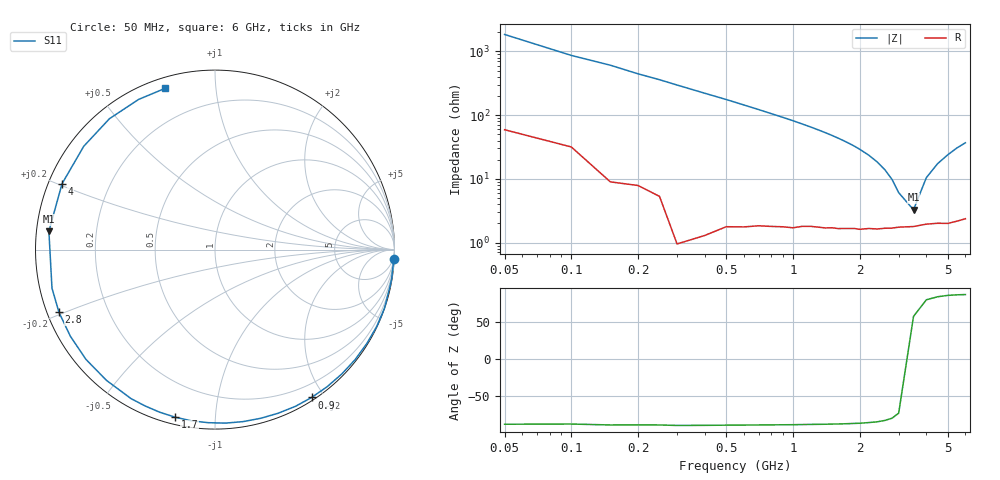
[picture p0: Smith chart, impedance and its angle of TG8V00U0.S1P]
! SIEMENS Discrete & RF Semiconductors
! BAT64
! Si Schottky Diode in SOT23
! VR = 8 V
! S-Parameters:  February  1997
# GHz  S  MA  R  50
!  f  S11
! GHz  MAG  ANG
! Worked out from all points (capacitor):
!   34 points, 50 MHz to 6 GHz, reference 50 ohm
!   read as one part to ground: C = 1.74 pF near 50 MHz
!   lowest |Z| = 3.28 ohm at 3.5 GHz (marker M1)
!   series resonance near 3.34 GHz, so ESL is about 1.3 nH
!   S11 on the Smith chart (normalised r, x): 50 MHz: 1, -37; 900 MHz: 0.04, -1.85; 1.7 GHz: 0.03, -0.79; 2.8 GHz: 0.03, -0.19; 4 GHz: 0.04, +0.21; 6 GHz: 0.05, +0.74
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0.05  0.9983 -3.1
0.1  0.9958 -6.6
0.15  0.9976 -9.4
0.25  0.996 -15.8
0.4  0.9975 -25.5
0.5  0.9947 -31.7
0.6  0.9925 -38.1
0.8  0.9869 -50.7
0.9  0.9841 -56.8
1  0.9816 -62.8
1.1  0.9772 -68.9
1.2  0.9737 -74.8
1.4  0.9686 -86.5
1.6  0.9629 -97.8
1.7  0.9597 -103.4
1.8  0.9569 -108.8
2  0.9529 -119.4
2.2  0.9468 -129.7
2.4  0.9439 -139.6
2.6  0.9394 -149.1
2.8  0.9369 -158.1
3  0.9333 -166.7
3.5  0.9311 173.7
4  0.9279 156.7
4.5  0.9306 141.8
5  0.9368 128.9
5.5  0.9387 117.0
6  0.9404 107.2
